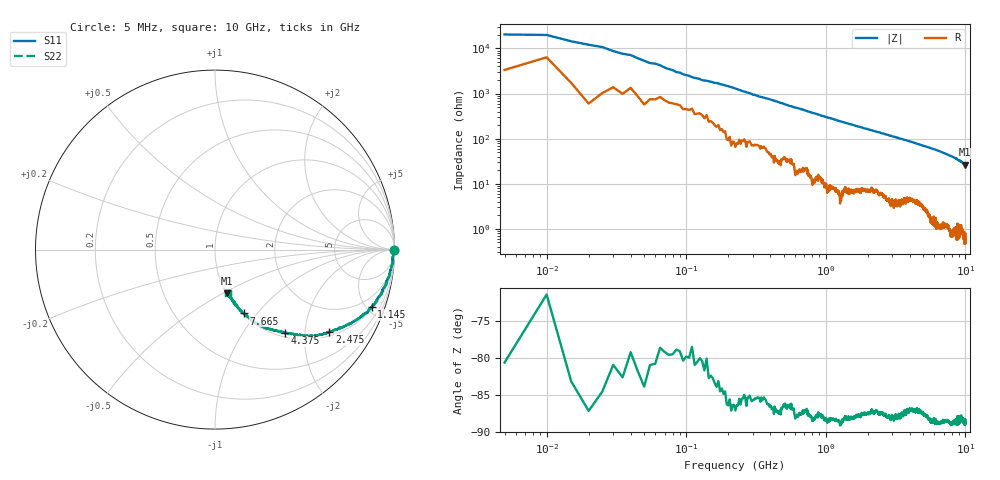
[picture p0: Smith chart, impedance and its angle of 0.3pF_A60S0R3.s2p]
! Amotech Co.,Ltd.
! http://www.amotech.co.kr/
! Part Number: A60S0R3
! These Parameters are Measured in Series Mode Connection
! Operation Temp=25[degC], DC Bias Voltage=0[V]
! Freq. Start=5[MHz] Stop=10[GHz], 2000[Steps]
! Date: Monday, July 13, 2020, 01:23:52
# GHZ S RI R 50.000000
!Freq.(Hz) S11(Real) S11(Imag) S21(Real) S21(Imag) S12(Real) S12(Imag) S22(Real) S22(Imag)
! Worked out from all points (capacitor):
!   2000 points, 5 MHz to 10 GHz, reference 50 ohm
!   read as one part in series: C = 618 fF near 55 MHz
!   lowest |Z| = 26.3 ohm at 9.995 GHz (marker M1)
!   S11 on the Smith chart (normalised r, x): 5 MHz: open; 1.145 GHz: 1.16, -5.40; 2.475 GHz: 1.12, -2.68; 4.375 GHz: 1.07, -1.58; 7.665 GHz: 1.02, -0.85; 10 GHz: 1.01, -0.53
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0.005  0.9992 -0.00481  0.000822 0.00481  0.000822 0.00481  0.9992 -0.00481
0.03  0.9981 -0.0112  0.00192 0.0112  0.00192 0.0112  0.9981 -0.0112
0.065  0.9948 -0.0229  0.00516 0.0229  0.00516 0.0229  0.9948 -0.0229
0.08  0.9936 -0.0293  0.00635 0.0293  0.00635 0.0293  0.9936 -0.0293
0.115  0.991 -0.0436  0.00896 0.0436  0.00896 0.0436  0.991 -0.0436
0.145  0.9905 -0.0521  0.00945 0.0521  0.00945 0.0521  0.9905 -0.0521
0.18  0.9898 -0.0612  0.0102 0.0612  0.0102 0.0612  0.9898 -0.0612
0.295  0.9826 -0.0996  0.0174 0.0996  0.0174 0.0996  0.9826 -0.0996
0.43  0.9717 -0.1386  0.0283 0.1386  0.0283 0.1386  0.9717 -0.1386
0.59  0.9518 -0.1883  0.0482 0.1883  0.0482 0.1883  0.9518 -0.1883
0.79  0.9277 -0.2418  0.0723 0.2418  0.0723 0.2418  0.9277 -0.2418
1.145  0.8721 -0.3195  0.1279 0.3195  0.1279 0.3195  0.8721 -0.3195
1.675  0.7725 -0.4008  0.2275 0.4008  0.2275 0.4008  0.7725 -0.4008
2.475  0.6376 -0.459  0.3624 0.459  0.3624 0.459  0.6376 -0.459
3.34  0.5103 -0.4797  0.4897 0.4797  0.4897 0.4797  0.5103 -0.4797
4.375  0.3909 -0.4651  0.6091 0.4651  0.6091 0.4651  0.3909 -0.4651
5.005  0.3302 -0.4493  0.6698 0.4493  0.6698 0.4493  0.3302 -0.4493
6.67  0.2123 -0.3986  0.7877 0.3986  0.7877 0.3986  0.2123 -0.3986
7.665  0.1599 -0.3555  0.8401 0.3555  0.8401 0.3555  0.1599 -0.3555
8.335  0.1302 -0.3269  0.8698 0.3269  0.8698 0.3269  0.1302 -0.3269
9.995  0.0683 -0.2437  0.9317 0.2437  0.9317 0.2437  0.0683 -0.2437
10  0.0698 -0.2438  0.9302 0.2438  0.9302 0.2438  0.0698 -0.2438
